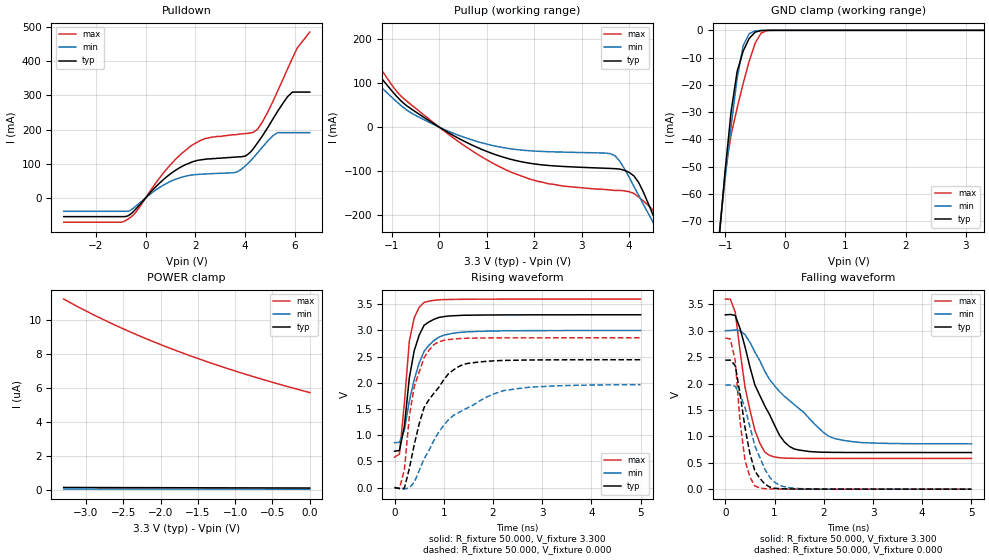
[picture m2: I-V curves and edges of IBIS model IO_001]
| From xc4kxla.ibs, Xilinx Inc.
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|   Model IO_001
[Model]   IO_001
Model_type   I/O
Polarity   Non-Inverting
Enable   Active-Low
Vinl =   0.800V
Vinh =   2.000V
Vmeas =   1.650V
Cref =  50.000pF
Rref =   1.000M
Vref =  0.000V
C_comp   7.300pF   5.500pF   8.800pF
[Temperature Range]   50.000   100.000   0.000
[Voltage Range]   3.300V   3.000V   3.600V
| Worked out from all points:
|   slope of the pulldown table from 0 to 0.495 V, typ, clamps not added: 12.8 ohm
|   slope of the pullup table from 0 to 0.495 V, typ, clamps not added: 16.3 ohm
|   GND clamp passes 1 mA (typ) near -0.52 V on its own axis
|   rising waveform, R_fixture 50.000, V_fixture 3.300: 20-80 % time 251ps typ, 353ps min, 189ps max; typ from 0.693 V to 3.3 V
|   rising waveform, R_fixture 50.000, V_fixture 0.000: 20-80 % time 599ps typ, 1.06ns min, 307ps max; typ from 0 V to 2.44 V
|   falling waveform, R_fixture 50.000, V_fixture 3.300: 20-80 % time 623ps typ, 1.14ns min, 333ps max; typ from 3.3 V to 0.694 V
|   falling waveform, R_fixture 50.000, V_fixture 0.000: 20-80 % time 284ps typ, 408ps min, 183ps max; typ from 2.44 V to 0.001 V
[Pulldown]
| voltage   I(typ)   I(min)   I(max)
-3.3V     -55.36mA   -39.74mA   -71.65mA
-900mV    -55.36mA   -39.74mA   -70.27mA
-400mV    -33.2mA    -24.66mA   -42.45mA
900mV     64.82mA    44.51mA    89.05mA
1.8V      103mA      66.09mA    151mA
3.6V      119mA      74.19mA    185mA
4V        122mA      93.03mA    188mA
4.5V      161mA      132mA      201mA
5.3V      253mA      191mA      312mA
5.7V      296mA      191mA      377mA
6.1V      310mA      191mA      440mA
6.6V      310mA      191mA      486mA
[Pullup]
| voltage   I(typ)   I(min)   I(max)
-3.3V     257mA      180mA      359mA
-2.3V     242mA      180mA      297mA
-1.9V     198mA      157mA      238mA
-700mV    49.86mA    40.16mA    60.72mA
400mV     -25mA      -18.17mA   -32.52mA
1.5V      -72.97mA   -49.19mA   -102mA
2.3V      -87.2mA    -55.86mA   -129mA
3.7V      -94.47mA   -64.95mA   -144mA
4.1V      -111mA     -135mA     -151mA
4.5V      -199mA     -216mA     -188mA
4.7V      -250mA     -255mA     -227mA
6.6V      -645mA     -572mA     -737mA
[GND_clamp]
| voltage   I(typ)   I(min)   I(max)
-3.3V     -539mA     -461mA     -635mA
-1.1V     -76.29mA   -74.81mA   -76.3mA
-1V       -51.66mA   -54.6mA    -52.25mA
-900mV    -29.77mA   -35.09mA   -38.23mA
-800mV    -15.1mA    -17.65mA   -28.49mA
-700mV    -7.645mA   -5.66mA    -19.53mA
-600mV    -2.968mA   -1.205mA   -11.34mA
-500mV    -649uA     -202uA     -4.68mA
-400mV    -83.34uA   -28.89uA   -976uA
-300mV    -8.303uA   -3.567uA   -95.2uA
3.3V      91.97nA    24.12nA    4.611uA
[POWER_clamp]
| voltage   I(typ)   I(min)   I(max)
-3.3V     126nA      27.84nA    11.23uA
-2.9V     121nA      27.69nA    10.3uA
-2.6V     117nA      27.29nA    9.671uA
-2.2V     113nA      27nA       8.903uA
-1.8V     109nA      25.98nA    8.207uA
-1.4V     104nA      25.34nA    7.571uA
-1V       101nA      24.85nA    6.988uA
-600mV    97.4nA     24.51nA    6.451uA
0V        91.96nA    23.79nA    5.718uA
[Ramp]
| variable   typ   min   max
dV/dt_r   1.464/0.573n   1.178/1.039n   1.715/0.326n
dV/dt_f   1.563/0.595n   1.285/1.118n   1.810/0.337n
R_load = 50.000
[Rising Waveform]
R_fixture = 50.000
V_fixture = 3.300
V_fixture_min = 3.000
V_fixture_max = 3.600
L_fixture = 0.000H
C_fixture = 0.000F
| time   V(typ)   V(min)   V(max)
0s        693mV      856mV      580mV
100ps     709mV      863mV      640mV
200ps     1.17V      1.093V     1.613V
300ps     2.091V     1.651V     2.793V
400ps     2.613V     2.06V      3.241V
500ps     2.907V     2.377V     3.44V
600ps     3.097V     2.598V     3.534V
900ps     3.247V     2.87V      3.584V
1.3ns     3.284V     2.959V     3.593V
5ns       3.298V     2.998V     3.598V
[Rising Waveform]
R_fixture = 50.000
V_fixture = 0.000
V_fixture_min = 0.000
V_fixture_max = 0.000
L_fixture = 0.000H
C_fixture = 0.000F
| time   V(typ)   V(min)   V(max)
0s        0V         0V         0V
100ps     -18.86mV   -12.02mV   -18.64mV
200ps     -12.29mV   -30.91mV   339mV
300ps     360mV      -5.003mV   1.351V
400ps     817mV      98.42mV    1.924V
600ps     1.527V     550mV      2.478V
800ps     1.8V       902mV      2.729V
1.4ns     2.354V     1.482V     2.847V
2.2ns     2.426V     1.848V     2.857V
5ns       2.44V      1.964V     2.859V
[Falling Waveform]
R_fixture = 50.000
V_fixture = 3.300
V_fixture_min = 3.000
V_fixture_max = 3.600
L_fixture = 0.000H
C_fixture = 0.000F
| time   V(typ)   V(min)   V(max)
0s        3.3V       3V         3.599V
100ps     3.308V     3.004V     3.597V
200ps     3.289V     3.016V     3.353V
400ps     2.692V     2.925V     1.926V
600ps     1.972V     2.597V     1.113V
800ps     1.578V     2.234V     703mV
900ps     1.409V     2.074V     639mV
1.3ns     811mV      1.681V     586mV
2.2ns     697mV      964mV      583mV
5ns       694mV      858mV      582mV
[Falling Waveform]
R_fixture = 50.000
V_fixture = 0.000
V_fixture_min = 0.000
V_fixture_max = 0.000
L_fixture = 0.000H
C_fixture = 0.000F
| time   V(typ)   V(min)   V(max)
0s        2.442V     1.97V      2.861V
100ps     2.444V     1.97V      2.844V
200ps     2.341V     1.948V     2.439V
300ps     1.796V     1.788V     1.264V
400ps     1.159V     1.543V     539mV
500ps     668mV      1.178V     229mV
600ps     345mV      818mV      60.81mV
900ps     41.86mV    228mV      6.693mV
1.2ns     7.356mV    46.11mV    2.836mV
5ns       1.142mV    1.206mV    1.066mV
